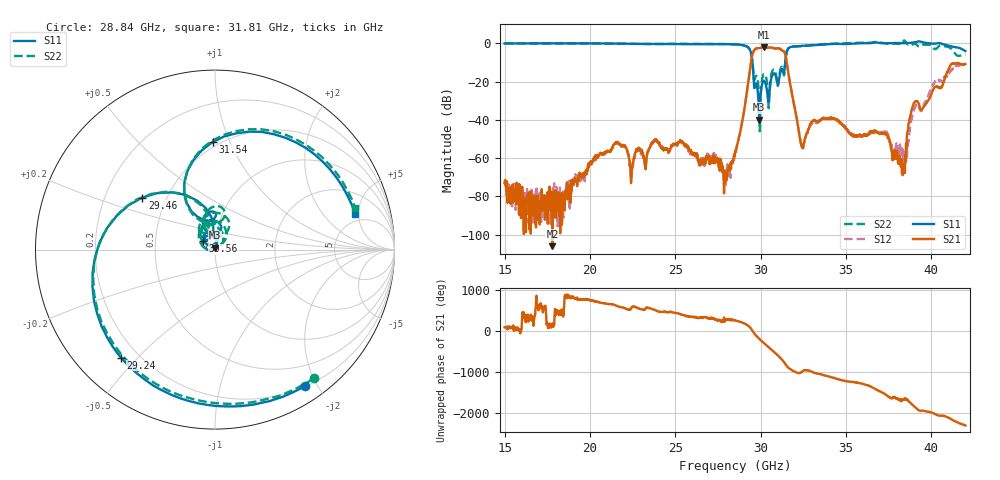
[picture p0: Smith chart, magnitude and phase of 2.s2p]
!The following data was pulled from an Agilent PNA
!This sNp file was generated from the data in the RF Test software
!NOTE:  Smoothing/Math/Corrections applied on any given trace ARE included in the data saved here
# MHz S dB R 50
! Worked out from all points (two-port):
!   1601 points, 15 GHz to 42 GHz, reference 50 ohm
!   highest |S21| = -2.17 dB at 30.17 GHz (marker M1); lowest = -105.9 dB at 17.8 GHz (marker M2)
!   |S21| within 3 dB of the highest: 29.54 GHz to 31.42 GHz (1.876 GHz wide, 6.16 % of centre)
!   lowest |S11| = -39.9 dB at 29.92 GHz (marker M3), VSWR 1.02, Z = 49.7 + j0.982 ohm
!   |S11| at or under -10 dB: 29.52 GHz to 31.44 GHz (1.921 GHz wide, 6.3 % of centre)
!   |S22| runs from -46.0 to 1.4 dB; largest |S21 - S12| = 0.095
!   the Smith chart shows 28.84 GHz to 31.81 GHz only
!   S11 on the Smith chart (normalised r, x): 28.84 GHz: 0.21, -1.84; 29.24 GHz: 0.14, -0.45; 29.46 GHz: 0.37, +0.28; 30.56 GHz: 0.87, +0.08; 31.54 GHz: 0.46, +0.86; 31.81 GHz: 4.05, +4.51
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15000  -0.17 17.8  -73.01 93.0  -73.59 99.6  -0.14 18.5
17801.25  -0.07 -35.8  -105.94 -170.3  -85.93 132.3  -0.10 -34.8
19505.62  -0.06 -73.6  -68.95 54.3  -69.71 24.3  -0.13 -73.2
24011.25  -0.43 159.3  -51.72 115.2  -52.00 120.0  -0.43 157.4
26593.12  -0.53 74.9  -61.14 -43.7  -64.61 -39.1  -0.37 74.3
28500  -0.60 -21.3  -57.09 -102.5  -57.20 -101.6  -0.59 -18.0
28837.5  -0.81 -56.5  -45.10 -139.5  -44.48 -140.3  -0.87 -52.4
29242.5  -1.96 -131.1  -22.40 141.5  -23.11 136.1  -2.03 -127.4
29461.88  -6.06 144.3  -8.37 46.2  -8.82 49.3  -5.69 147.6
29917.5  -39.86 103.9  -2.53 172.0  -2.52 173.0  -29.47 33.5
30170.62  -19.61 119.6  -2.17 74.3  -2.17 76.3  -16.21 110.2
30558.75  -21.84 144.9  -2.22 -64.7  -2.24 -63.5  -20.71 143.4
31081.88  -18.84 115.9  -2.81 99.6  -2.59 100.0  -17.70 113.8
31537.5  -4.45 91.3  -10.41 -130.8  -10.18 -134.2  -4.35 91.7
31807.5  -1.89 14.2  -24.72 136.3  -25.33 135.8  -1.78 16.7
32415  -1.40 -107.4  -53.91 91.5  -54.13 84.9  -1.61 -105.4
33005.62  -1.10 176.8  -41.15 92.2  -41.76 91.2  -1.02 176.1
34490.62  -0.35 94.5  -39.97 -85.0  -40.13 -81.4  -0.12 92.7
37511.25  -0.01 25.9  -49.92 -154.7  -48.01 -143.6  -0.31 22.7
38355  0.00 11.6  -66.01 140.3  -59.03 52.5  0.86 12.3
39013.12  0.45 1.3  -30.98 -37.1  -33.70 -19.9  -0.25 -2.6
42000  -4.09 -80.7  -10.86 -133.5  -10.85 -127.1  -5.91 -50.3
